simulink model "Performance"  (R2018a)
settings: Solver=ode113  StartTime=0.0  StopTime=20  FixedStep=0.0001  RelTol=1e-5  EnableMultiTasking=on
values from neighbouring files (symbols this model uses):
  d2r = pi/180    (= 0.0174532925199)    [init.m]
  Kr = Kq; Kr(3:4)=-Kq(3:4)    [init.m]
  r2d = 1/d2r    (= 57.2957795131)    [init.m]
  Wf = 20    [init.m]
undefined symbols (not defined in the file or in its folder): Aa, Av, Ba, Bv, Ca, Cv, Da, Dv, Kq, TVC

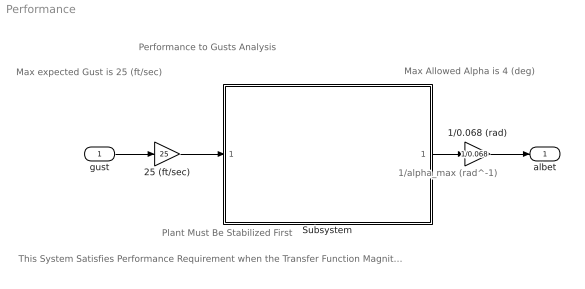
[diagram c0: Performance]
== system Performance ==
  note: Performance to Gusts Analysis
  note: Plant Must Be Stabilized First
  note: Max expected Gust is 25 (ft/sec)
  note: 1/alpha_max (rad^-1)
  note: This System Satisfies Performance Requirement when the Transfer Function Magnitude is Less than One at All Frequencies
  note: Max Allowed Alpha is 4 (deg)
  gust : Inport
  1/0.068 (rad) : Gain  Gain=1/0.068
  25 (ft/sec) : Gain  Gain=25
  Subsystem : Subsystem
  albet : Outport
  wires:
  gust/1 -> 25 (ft/sec)/1
  Subsystem/1(albet) -> 1/0.068 (rad)/1
  25 (ft/sec)/1 -> Subsystem/1(gust)
  1/0.068 (rad)/1 -> albet/1

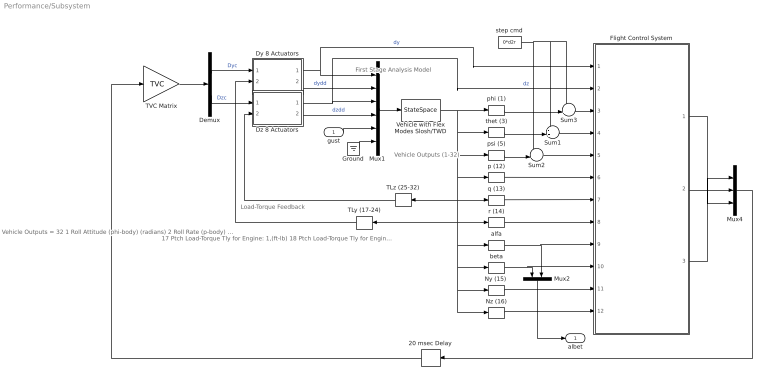
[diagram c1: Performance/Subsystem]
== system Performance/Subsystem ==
  note: First Stage Analysis Model
  note: Load-Torque Feedback
  note: 17 Ptch Load-Torque Tly for Engine: 1,(ft-lb) 18 Ptch Load-Torque Tly for Engine: 2,(ft-lb) 19 Ptch Load-Torque Tly for Engine: 3,(ft-lb) 20 Ptch Load-Torque Tly for Engine: 4,(ft-lb) 21 Ptch Load-Torque Tly for Engine: 5,(ft-lb) 22 Ptch Load-Torque Tly for Engine: 6,(ft-lb) 23 Ptch Load-Torque Tly for Engine: 7,(ft-lb) 24 Ptch Load-Torque Tly for Engine: 8,(ft-lb) 25 Yaw Load-Torque Tlz for Engine: 1,(ft-lb) 26 Yaw Load-Torque Tlz for Engine: 2,(ft-lb) 27 Yaw Load-Torque Tlz for Engine: 3,(ft-lb) 28 Yaw Load-Torque Tlz for Engine: 4,(ft-lb) 29 Yaw Load-Torque Tlz for Engine: 5,(ft-lb) 30 Yaw Load-Torque Tlz for Engine: 6,(ft-lb) 31 Yaw Load-Torque Tlz for Engine: 7,(ft-lb) 32 Yaw Load-Torque Tlz for Engine: 8,(ft-lb)
  note: Vehicle Outputs = 32 1 Roll Attitude (phi-body) (radians) 2 Roll Rate (p-body) (rad/sec) 3 Pitch Attitude (thet-bdy) (radians) 4 Pitch Rate (q-body) (rad/sec) 5 Yaw Attitude (psi-body) (radians) 6 Yaw Rate (r-body) (rad/sec) 7 Angle of attack, alfa, (radians) 8 Angle of sideslip, beta, (radian) 9 Change in Altitude, delta-h, (feet) 10 Forward Acceleration (V-dot) (ft/sec) 11 Cross Range Velocity (Vcr) (ft/sec) 12 Rate-Gyro # 1, Roll Rate (Body) (rad/sec) 13 Rate-Gyro # 2, Pitch Rate (Body) (rad/sec) 14 Rate-Gyro # 3, Yaw Rate (Body) (rad/sec) 15 Accelerom # 1, (along Y), (ft/sec^2) Translat. Accelerat. 16 Accelerom # 2, (along Z), (ft/sec^2) Translat. Accelerat.
  note: Vehicle Outputs (1-32)
  gust : Inport
  20 msec Delay : TransportDelay  DelayTime="[1  1  1]*0.02"  InitialOutput="[0  0  0]"  PadeOrder=2
  Demux : Demux  Outputs=[8, 8]
  Dy 8 Actuators : Subsystem
  Dz 8 Actuators : Subsystem
  Flight Control System : Subsystem
  Ground : Ground
  Mux1 : Mux  Inputs=[8, 8, 8, 8, 1, 38]
  Mux2 : Mux  Inputs=2
  Mux4 : Mux  Inputs=3
  "Ny (15) " : Selector  InputPortWidth=70  IndexOptions=Index vector (dialog)  Indices=[15]  OutputSizes=1
  Nz (16) : Selector  InputPortWidth=70  IndexOptions=Index vector (dialog)  Indices=[16]  OutputSizes=1
  Sum1 : Sum  Inputs=-+|
  Sum2 : Sum  Inputs=-+|
  Sum3 : Sum  Inputs=-+|
  TLy (17-24) : Selector  InputPortWidth=70  IndexOptions=Index vector (dialog)  Indices=[17:24]  OutputSizes=1
  TLz (25-32) : Selector  InputPortWidth=70  IndexOptions=Index vector (dialog)  Indices=[25:32]  OutputSizes=1
  TVC Matrix : Gain  Gain=TVC  Multiplication=Matrix(K*u)
  Vehicle with Flex Modes Slosh/TWD : StateSpace  A=Av  B=Bv  C=Cv  D=Dv  InitialCondition=0
  alfa : Selector  InputPortWidth=70  IndexOptions=Index vector (dialog)  Indices=[7]  OutputSizes=1
  beta : Selector  InputPortWidth=70  IndexOptions=Index vector (dialog)  Indices=[8]  OutputSizes=1
  p (12) : Selector  InputPortWidth=70  IndexOptions=Index vector (dialog)  Indices=[12]  OutputSizes=1
  phi (1) : Selector  InputPortWidth=70  IndexOptions=Index vector (dialog)  Indices=[1]  OutputSizes=1
  psi (5) : Selector  InputPortWidth=70  IndexOptions=Index vector (dialog)  Indices=[5]  OutputSizes=1
  q (13) : Selector  InputPortWidth=70  IndexOptions=Index vector (dialog)  Indices=[13]  OutputSizes=1
  r (14) : Selector  InputPortWidth=70  IndexOptions=Index vector (dialog)  Indices=[14]  OutputSizes=1
  step cmd : Constant  Value=0*d2r
  thet (3) : Selector  InputPortWidth=70  IndexOptions=Index vector (dialog)  Indices=[3]  OutputSizes=1
  albet : Outport
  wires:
  Mux1/1 -> Vehicle with Flex Modes Slosh/TWD/1
  Dz 8 Actuators/2(dzdd) -> Mux1/4  "dzdd"
  p (12)/1 -> Flight Control System/6(p)
  Vehicle with Flex Modes Slosh/TWD/1 -> TLz (25-32)/1, "Ny (15) "/1, Nz (16)/1, beta/1, alfa/1, TLy (17-24)/1, r (14)/1, q (13)/1, p (12)/1, psi (5)/1, thet (3)/1, phi (1)/1
  20 msec Delay/1 -> TVC Matrix/1
  TVC Matrix/1 -> Demux/1
  "Ny (15) "/1 -> Flight Control System/11(NY)
  Dz 8 Actuators/1(dz) -> Flight Control System/2(dz), Mux1/3  "dz"
  r (14)/1 -> Flight Control System/8(r)
  step cmd/1 -> Sum1/1, Sum3/1, Sum2/1
  TLy (17-24)/1 -> Dy 8 Actuators/2(TLy)
  TLz (25-32)/1 -> Dz 8 Actuators/2(TLz)
  alfa/1 -> Flight Control System/9(alfa), Mux2/2
  Flight Control System/2(DQ_tvc) -> Mux4/2
  Flight Control System/1(DP_tvc) -> Mux4/1
  Dy 8 Actuators/1(dy) -> Flight Control System/1(dy), Mux1/1  "dy"
  q (13)/1 -> Flight Control System/7(q)
  Dy 8 Actuators/2(dydd) -> Mux1/2  "dydd"
  beta/1 -> Flight Control System/10(beta), Mux2/1
  Flight Control System/3(DR_tvc) -> Mux4/3
  psi (5)/1 -> Sum2/2
  Demux/2 -> Dz 8 Actuators/1(dzc)  "Dzc"
  Sum2/1 -> Flight Control System/5(psi)
  Sum3/1 -> Flight Control System/3(phi)
  Sum1/1 -> Flight Control System/4(thet)
  Nz (16)/1 -> Flight Control System/12(NZ)
  thet (3)/1 -> Sum1/2
  Demux/1 -> Dy 8 Actuators/1(dyc)  "Dyc"
  phi (1)/1 -> Sum3/2
  Mux4/1 -> 20 msec Delay/1
  Ground/1 -> Mux1/6
  gust/1 -> Mux1/5
  Mux2/1 -> albet/1

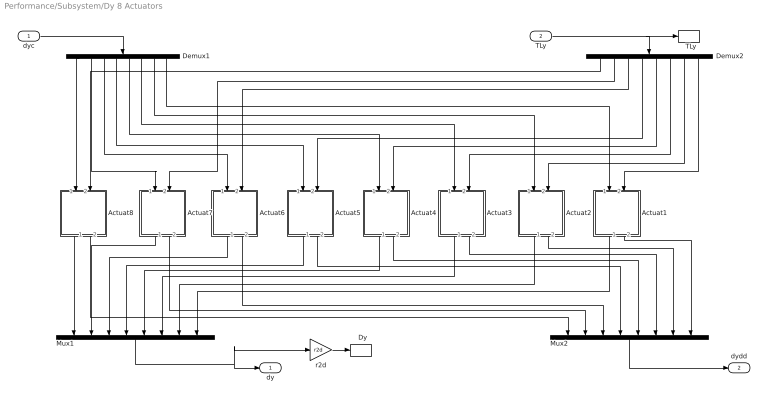
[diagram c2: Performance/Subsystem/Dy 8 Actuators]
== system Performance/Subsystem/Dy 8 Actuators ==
  dyc : Inport
  TLy : Inport  Port=2
  "  Dy" : ToWorkspace  VariableName=DY  SampleTime=-1
  "  TLy" : ToWorkspace  VariableName=TLy  SampleTime=-1
  Actuat1 : Subsystem
  Actuat2 : Subsystem
  Actuat3 : Subsystem
  Actuat4 : Subsystem
  Actuat5 : Subsystem
  Actuat6 : Subsystem
  Actuat7 : Subsystem
  Actuat8 : Subsystem
  Demux1 : Demux  Outputs=8
  Demux2 : Demux  Outputs=8
  Mux1 : Mux  Inputs=8
  Mux2 : Mux  Inputs=8
  r2d : Gain  Gain=r2d
  dy : Outport
  dydd : Outport  Port=2
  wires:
  TLy/1 -> "  TLy"/1, Demux2/1
  Mux2/1 -> dydd/1
  Actuat5/1(dout) -> Mux1/4
  Demux1/5 -> Actuat4/1(delin)
  Actuat3/2(ddot) -> Mux2/6
  Actuat8/1(dout) -> Mux1/1
  Demux1/4 -> Actuat5/1(delin)
  Actuat1/1(dout) -> Mux1/8
  Actuat4/2(ddot) -> Mux2/5
  Actuat4/1(dout) -> Mux1/5
  Demux2/4 -> Actuat5/2(TL)
  Demux2/6 -> Actuat3/2(TL)
  Demux2/7 -> Actuat2/2(TL)
  Actuat6/2(ddot) -> Mux2/3
  Demux2/2 -> Actuat7/2(TL)
  Actuat5/2(ddot) -> Mux2/4
  Demux1/3 -> Actuat6/1(delin)
  Actuat2/2(ddot) -> Mux2/7
  Actuat8/2(ddot) -> Mux2/1
  dyc/1 -> Demux1/1
  Mux1/1 -> r2d/1, dy/1
  Actuat1/2(ddot) -> Mux2/8
  Actuat7/2(ddot) -> Mux2/2
  Demux1/2 -> Actuat7/1(delin)
  Demux1/7 -> Actuat2/1(delin)
  Demux1/8 -> Actuat1/1(delin)
  Actuat7/1(dout) -> Mux1/2
  Demux2/5 -> Actuat4/2(TL)
  Demux1/1 -> Actuat8/1(delin)
  Demux2/1 -> Actuat8/2(TL)
  Actuat2/1(dout) -> Mux1/7
  Demux2/8 -> Actuat1/2(TL)
  Demux2/3 -> Actuat6/2(TL)
  Actuat3/1(dout) -> Mux1/6
  Actuat6/1(dout) -> Mux1/3
  Demux1/6 -> Actuat3/1(delin)
  r2d/1 -> "  Dy"/1

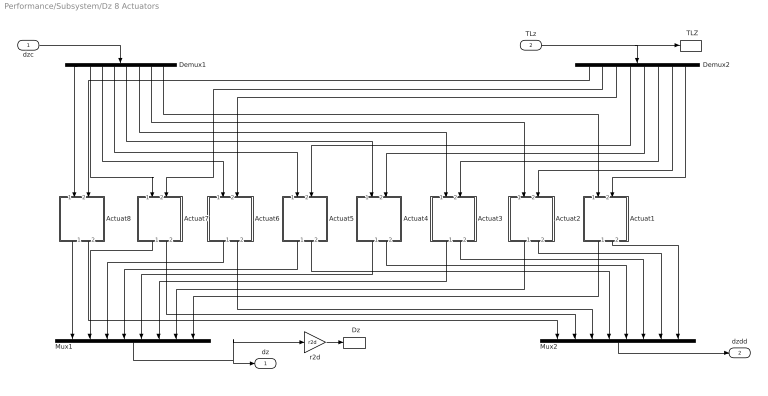
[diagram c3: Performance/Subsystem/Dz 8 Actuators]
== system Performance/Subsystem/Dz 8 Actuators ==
  dzc : Inport
  TLz : Inport  Port=2
  "  Dz" : ToWorkspace  VariableName=DZ  SampleTime=-1
  "  TLZ" : ToWorkspace  VariableName=TLz  SampleTime=-1
  Actuat1 : Subsystem
  Actuat2 : Subsystem
  Actuat3 : Subsystem
  Actuat4 : Subsystem
  Actuat5 : Subsystem
  Actuat6 : Subsystem
  Actuat7 : Subsystem
  Actuat8 : Subsystem
  Demux1 : Demux  Outputs=8
  Demux2 : Demux  Outputs=8
  Mux1 : Mux  Inputs=8
  Mux2 : Mux  Inputs=8
  r2d : Gain  Gain=r2d
  dz : Outport
  dzdd : Outport  Port=2
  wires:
  TLz/1 -> "  TLZ"/1, Demux2/1
  Mux2/1 -> dzdd/1
  Actuat5/1(dout) -> Mux1/4
  Demux1/5 -> Actuat4/1(delin)
  Actuat3/2(ddot) -> Mux2/6
  Actuat8/1(dout) -> Mux1/1
  Demux1/4 -> Actuat5/1(delin)
  Actuat1/1(dout) -> Mux1/8
  Actuat4/2(ddot) -> Mux2/5
  Actuat4/1(dout) -> Mux1/5
  Demux2/4 -> Actuat5/2(TL)
  Demux2/6 -> Actuat3/2(TL)
  Demux2/7 -> Actuat2/2(TL)
  Actuat6/2(ddot) -> Mux2/3
  Demux2/2 -> Actuat7/2(TL)
  Actuat5/2(ddot) -> Mux2/4
  Demux1/3 -> Actuat6/1(delin)
  Actuat2/2(ddot) -> Mux2/7
  Actuat8/2(ddot) -> Mux2/1
  dzc/1 -> Demux1/1
  Mux1/1 -> r2d/1, dz/1
  Actuat1/2(ddot) -> Mux2/8
  Actuat7/2(ddot) -> Mux2/2
  Demux1/2 -> Actuat7/1(delin)
  Demux1/7 -> Actuat2/1(delin)
  Demux1/8 -> Actuat1/1(delin)
  Actuat7/1(dout) -> Mux1/2
  Demux2/5 -> Actuat4/2(TL)
  Demux1/1 -> Actuat8/1(delin)
  Demux2/1 -> Actuat8/2(TL)
  Actuat2/1(dout) -> Mux1/7
  Demux2/8 -> Actuat1/2(TL)
  Demux2/3 -> Actuat6/2(TL)
  Actuat3/1(dout) -> Mux1/6
  Actuat6/1(dout) -> Mux1/3
  Demux1/6 -> Actuat3/1(delin)
  r2d/1 -> "  Dz"/1

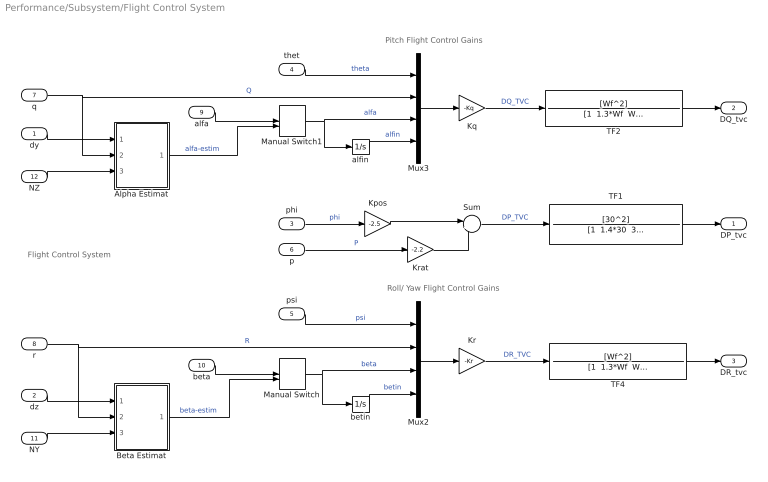
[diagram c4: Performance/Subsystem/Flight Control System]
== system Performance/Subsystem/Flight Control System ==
  note: Flight Control System
  note: Roll/ Yaw Flight Control Gains
  note: Pitch Flight Control Gains
  dy : Inport
  dz : Inport  Port=2
  phi : Inport  Port=3
  thet : Inport  Port=4
  psi : Inport  Port=5
  p : Inport  Port=6
  q : Inport  Port=7
  r : Inport  Port=8
  alfa : Inport  Port=9
  beta : Inport  Port=10
  NY : Inport  Port=11
  NZ : Inport  Port=12
  Alpha Estimat : Subsystem
  Beta Estimat : Subsystem
  Kpos : Gain  Gain=-2.5  Multiplication=Matrix(K*u)
  Kq : Gain  Gain=-Kq  Multiplication=Matrix(K*u)
  Kr : Gain  Gain=-Kr  Multiplication=Matrix(K*u)
  Krat : Gain  Gain=-2.2  Multiplication=Matrix(K*u)
  Manual Switch : ManualSwitch  CurrentSetting=0
  Manual Switch1 : ManualSwitch  CurrentSetting=0
  Mux2 : Mux
  Mux3 : Mux
  Sum : Sum  Inputs=|++
  TF1 : TransferFcn  Numerator=[30^2]  Denominator="[1  1.4*30  30^2]"
  TF2 : TransferFcn  Numerator=[Wf^2]  Denominator="[1  1.3*Wf  Wf^2]"
  TF4 : TransferFcn  Numerator=[Wf^2]  Denominator="[1  1.3*Wf  Wf^2]"
  alfin : Integrator
  betin : Integrator
  DP_tvc : Outport
  DQ_tvc : Outport  Port=2
  DR_tvc : Outport  Port=3
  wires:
  TF4/1 -> DR_tvc/1
  Kr/1 -> TF4/1  "DR_TVC"
  TF2/1 -> DQ_tvc/1
  TF1/1 -> DP_tvc/1
  Mux2/1 -> Kr/1
  phi/1 -> Kpos/1  "phi"
  p/1 -> Krat/1  "P"
  Krat/1 -> Sum/2
  Sum/1 -> TF1/1  "DP_TVC"
  Kpos/1 -> Sum/1
  Mux3/1 -> Kq/1
  dz/1 -> Beta Estimat/1(dz)
  dy/1 -> Alpha Estimat/1(dy)
  Beta Estimat/1(betest) -> Manual Switch/2  "beta-estim"
  NY/1 -> Beta Estimat/3(Ydd)
  NZ/1 -> Alpha Estimat/3(Zdd)
  Kq/1 -> TF2/1  "DQ_TVC"
  thet/1 -> Mux3/1  "theta"
  alfin/1 -> Mux3/4  "alfin"
  r/1 -> Beta Estimat/2(r), Mux2/2  "R"
  q/1 -> Mux3/2, Alpha Estimat/2(q)  "Q"
  betin/1 -> Mux2/4  "betin"
  psi/1 -> Mux2/1  "psi"
  Manual Switch/1 -> Mux2/3, betin/1  "beta"
  beta/1 -> Manual Switch/1
  Manual Switch1/1 -> alfin/1, Mux3/3  "alfa"
  alfa/1 -> Manual Switch1/1
  Alpha Estimat/1(alfest) -> Manual Switch1/2  "alfa-estim"

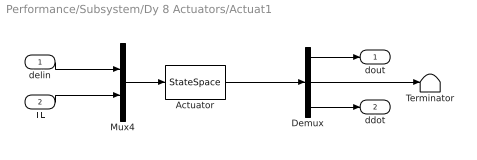
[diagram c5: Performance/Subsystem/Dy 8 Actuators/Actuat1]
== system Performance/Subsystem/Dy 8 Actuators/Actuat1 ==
  delin : Inport
  TL : Inport  Port=2
  Actuator : StateSpace  A=Aa  B=Ba  C=Ca  D=Da  InitialCondition=0
  Demux : Demux  Outputs=3
  Mux4 : Mux  Inputs=2
  Terminator : Terminator
  dout : Outport
  ddot : Outport  Port=2
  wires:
  Demux/3 -> ddot/1
  TL/1 -> Mux4/2
  Mux4/1 -> Actuator/1
  Actuator/1 -> Demux/1
  delin/1 -> Mux4/1
  Demux/1 -> dout/1
  Demux/2 -> Terminator/1

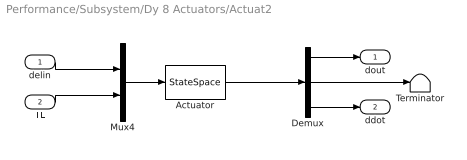
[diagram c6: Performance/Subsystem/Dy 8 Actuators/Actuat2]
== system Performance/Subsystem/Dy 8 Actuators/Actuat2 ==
  delin : Inport
  TL : Inport  Port=2
  Actuator : StateSpace  A=Aa  B=Ba  C=Ca  D=Da  InitialCondition=0
  Demux : Demux  Outputs=3
  Mux4 : Mux  Inputs=2
  Terminator : Terminator
  dout : Outport
  ddot : Outport  Port=2
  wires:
  Demux/3 -> ddot/1
  TL/1 -> Mux4/2
  Mux4/1 -> Actuator/1
  Actuator/1 -> Demux/1
  delin/1 -> Mux4/1
  Demux/1 -> dout/1
  Demux/2 -> Terminator/1

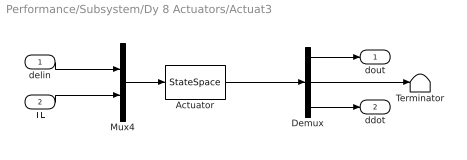
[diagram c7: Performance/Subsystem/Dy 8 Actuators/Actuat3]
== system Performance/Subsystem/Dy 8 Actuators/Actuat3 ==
  delin : Inport
  TL : Inport  Port=2
  Actuator : StateSpace  A=Aa  B=Ba  C=Ca  D=Da  InitialCondition=0
  Demux : Demux  Outputs=3
  Mux4 : Mux  Inputs=2
  Terminator : Terminator
  dout : Outport
  ddot : Outport  Port=2
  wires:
  Demux/3 -> ddot/1
  TL/1 -> Mux4/2
  Mux4/1 -> Actuator/1
  Actuator/1 -> Demux/1
  delin/1 -> Mux4/1
  Demux/1 -> dout/1
  Demux/2 -> Terminator/1

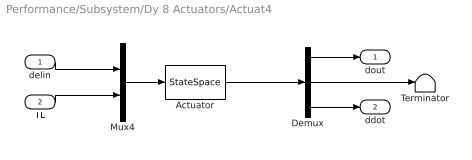
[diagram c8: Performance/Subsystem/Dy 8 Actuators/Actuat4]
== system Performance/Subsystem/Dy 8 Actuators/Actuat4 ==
  delin : Inport
  TL : Inport  Port=2
  Actuator : StateSpace  A=Aa  B=Ba  C=Ca  D=Da  InitialCondition=0
  Demux : Demux  Outputs=3
  Mux4 : Mux  Inputs=2
  Terminator : Terminator
  dout : Outport
  ddot : Outport  Port=2
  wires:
  Demux/3 -> ddot/1
  TL/1 -> Mux4/2
  Mux4/1 -> Actuator/1
  Actuator/1 -> Demux/1
  delin/1 -> Mux4/1
  Demux/1 -> dout/1
  Demux/2 -> Terminator/1

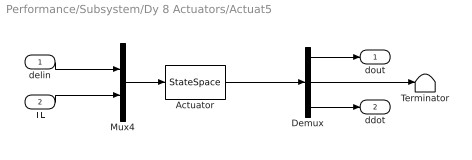
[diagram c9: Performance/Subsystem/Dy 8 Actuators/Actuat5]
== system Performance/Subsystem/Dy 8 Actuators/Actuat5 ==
  delin : Inport
  TL : Inport  Port=2
  Actuator : StateSpace  A=Aa  B=Ba  C=Ca  D=Da  InitialCondition=0
  Demux : Demux  Outputs=3
  Mux4 : Mux  Inputs=2
  Terminator : Terminator
  dout : Outport
  ddot : Outport  Port=2
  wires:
  Demux/3 -> ddot/1
  TL/1 -> Mux4/2
  Mux4/1 -> Actuator/1
  Actuator/1 -> Demux/1
  delin/1 -> Mux4/1
  Demux/1 -> dout/1
  Demux/2 -> Terminator/1

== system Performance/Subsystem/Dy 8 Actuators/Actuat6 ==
  delin : Inport
  TL : Inport  Port=2
  Actuator : StateSpace  A=Aa  B=Ba  C=Ca  D=Da  InitialCondition=0
  Demux : Demux  Outputs=3
  Mux4 : Mux  Inputs=2
  Terminator : Terminator
  dout : Outport
  ddot : Outport  Port=2
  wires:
  Demux/3 -> ddot/1
  TL/1 -> Mux4/2
  Mux4/1 -> Actuator/1
  Actuator/1 -> Demux/1
  delin/1 -> Mux4/1
  Demux/1 -> dout/1
  Demux/2 -> Terminator/1

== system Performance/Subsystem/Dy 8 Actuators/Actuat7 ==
  delin : Inport
  TL : Inport  Port=2
  Actuator : StateSpace  A=Aa  B=Ba  C=Ca  D=Da  InitialCondition=0
  Demux : Demux  Outputs=3
  Mux4 : Mux  Inputs=2
  Terminator : Terminator
  dout : Outport
  ddot : Outport  Port=2
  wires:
  Demux/3 -> ddot/1
  TL/1 -> Mux4/2
  Mux4/1 -> Actuator/1
  Actuator/1 -> Demux/1
  delin/1 -> Mux4/1
  Demux/1 -> dout/1
  Demux/2 -> Terminator/1

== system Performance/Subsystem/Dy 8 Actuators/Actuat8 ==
  delin : Inport
  TL : Inport  Port=2
  Actuator : StateSpace  A=Aa  B=Ba  C=Ca  D=Da  InitialCondition=0
  Demux : Demux  Outputs=3
  Mux4 : Mux  Inputs=2
  Terminator : Terminator
  dout : Outport
  ddot : Outport  Port=2
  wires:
  Demux/3 -> ddot/1
  TL/1 -> Mux4/2
  Mux4/1 -> Actuator/1
  Actuator/1 -> Demux/1
  delin/1 -> Mux4/1
  Demux/1 -> dout/1
  Demux/2 -> Terminator/1

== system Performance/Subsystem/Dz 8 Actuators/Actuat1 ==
  delin : Inport
  TL : Inport  Port=2
  Actuator : StateSpace  A=Aa  B=Ba  C=Ca  D=Da  InitialCondition=0
  Demux : Demux  Outputs=3
  Mux4 : Mux  Inputs=2
  Terminator : Terminator
  dout : Outport
  ddot : Outport  Port=2
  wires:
  Demux/3 -> ddot/1
  TL/1 -> Mux4/2
  Mux4/1 -> Actuator/1
  Actuator/1 -> Demux/1
  delin/1 -> Mux4/1
  Demux/1 -> dout/1
  Demux/2 -> Terminator/1

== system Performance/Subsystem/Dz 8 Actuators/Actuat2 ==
  delin : Inport
  TL : Inport  Port=2
  Actuator : StateSpace  A=Aa  B=Ba  C=Ca  D=Da  InitialCondition=0
  Demux : Demux  Outputs=3
  Mux4 : Mux  Inputs=2
  Terminator : Terminator
  dout : Outport
  ddot : Outport  Port=2
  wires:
  Demux/3 -> ddot/1
  TL/1 -> Mux4/2
  Mux4/1 -> Actuator/1
  Actuator/1 -> Demux/1
  delin/1 -> Mux4/1
  Demux/1 -> dout/1
  Demux/2 -> Terminator/1

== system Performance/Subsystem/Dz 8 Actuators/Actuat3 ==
  delin : Inport
  TL : Inport  Port=2
  Actuator : StateSpace  A=Aa  B=Ba  C=Ca  D=Da  InitialCondition=0
  Demux : Demux  Outputs=3
  Mux4 : Mux  Inputs=2
  Terminator : Terminator
  dout : Outport
  ddot : Outport  Port=2
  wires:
  Demux/3 -> ddot/1
  TL/1 -> Mux4/2
  Mux4/1 -> Actuator/1
  Actuator/1 -> Demux/1
  delin/1 -> Mux4/1
  Demux/1 -> dout/1
  Demux/2 -> Terminator/1

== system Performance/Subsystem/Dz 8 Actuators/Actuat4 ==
  delin : Inport
  TL : Inport  Port=2
  Actuator : StateSpace  A=Aa  B=Ba  C=Ca  D=Da  InitialCondition=0
  Demux : Demux  Outputs=3
  Mux4 : Mux  Inputs=2
  Terminator : Terminator
  dout : Outport
  ddot : Outport  Port=2
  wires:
  Demux/3 -> ddot/1
  TL/1 -> Mux4/2
  Mux4/1 -> Actuator/1
  Actuator/1 -> Demux/1
  delin/1 -> Mux4/1
  Demux/1 -> dout/1
  Demux/2 -> Terminator/1

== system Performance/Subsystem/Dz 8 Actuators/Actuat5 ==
  delin : Inport
  TL : Inport  Port=2
  Actuator : StateSpace  A=Aa  B=Ba  C=Ca  D=Da  InitialCondition=0
  Demux : Demux  Outputs=3
  Mux4 : Mux  Inputs=2
  Terminator : Terminator
  dout : Outport
  ddot : Outport  Port=2
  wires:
  Demux/3 -> ddot/1
  TL/1 -> Mux4/2
  Mux4/1 -> Actuator/1
  Actuator/1 -> Demux/1
  delin/1 -> Mux4/1
  Demux/1 -> dout/1
  Demux/2 -> Terminator/1

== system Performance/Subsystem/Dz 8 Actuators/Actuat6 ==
  delin : Inport
  TL : Inport  Port=2
  Actuator : StateSpace  A=Aa  B=Ba  C=Ca  D=Da  InitialCondition=0
  Demux : Demux  Outputs=3
  Mux4 : Mux  Inputs=2
  Terminator : Terminator
  dout : Outport
  ddot : Outport  Port=2
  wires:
  Demux/3 -> ddot/1
  TL/1 -> Mux4/2
  Mux4/1 -> Actuator/1
  Actuator/1 -> Demux/1
  delin/1 -> Mux4/1
  Demux/1 -> dout/1
  Demux/2 -> Terminator/1

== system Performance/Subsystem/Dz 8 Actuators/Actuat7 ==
  delin : Inport
  TL : Inport  Port=2
  Actuator : StateSpace  A=Aa  B=Ba  C=Ca  D=Da  InitialCondition=0
  Demux : Demux  Outputs=3
  Mux4 : Mux  Inputs=2
  Terminator : Terminator
  dout : Outport
  ddot : Outport  Port=2
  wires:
  Demux/3 -> ddot/1
  TL/1 -> Mux4/2
  Mux4/1 -> Actuator/1
  Actuator/1 -> Demux/1
  delin/1 -> Mux4/1
  Demux/1 -> dout/1
  Demux/2 -> Terminator/1

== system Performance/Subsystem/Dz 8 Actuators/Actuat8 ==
  delin : Inport
  TL : Inport  Port=2
  Actuator : StateSpace  A=Aa  B=Ba  C=Ca  D=Da  InitialCondition=0
  Demux : Demux  Outputs=3
  Mux4 : Mux  Inputs=2
  Terminator : Terminator
  dout : Outport
  ddot : Outport  Port=2
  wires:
  Demux/3 -> ddot/1
  TL/1 -> Mux4/2
  Mux4/1 -> Actuator/1
  Actuator/1 -> Demux/1
  delin/1 -> Mux4/1
  Demux/1 -> dout/1
  Demux/2 -> Terminator/1

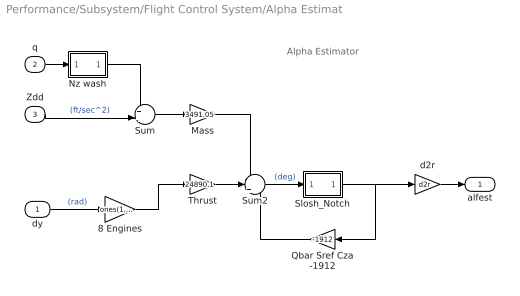
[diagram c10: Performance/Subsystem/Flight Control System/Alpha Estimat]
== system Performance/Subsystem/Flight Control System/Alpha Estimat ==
  note: Alpha Estimator
  dy : Inport
  q : Inport  Port=2
  Zdd : Inport  Port=3
  8 Engines : Gain  Gain=ones(1,8)  Multiplication=Matrix(K*u) (u vector)
  Mass : Gain  Gain=3491.05
  Nz wash : Subsystem
  Qbar Sref Cza -1912 : Gain  Gain=-1912
  Slosh_Notch : Subsystem
  Sum : Sum  Inputs=++|
  Sum2 : Sum  Inputs=--+
  Thrust : Gain  Gain=24890.1
  d2r : Gain  Gain=d2r
  alfest : Outport
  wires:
  8 Engines/1 -> Thrust/1
  Thrust/1 -> Sum2/2
  Mass/1 -> Sum2/1
  Slosh_Notch/1(ou) -> Qbar Sref Cza -1912/1, d2r/1
  Nz wash/1(ou) -> Sum/1
  Sum2/1 -> Slosh_Notch/1(in)  "(deg)"
  Qbar Sref Cza -1912/1 -> Sum2/3
  Zdd/1 -> Sum/2  "(ft/sec^2)"
  d2r/1 -> alfest/1
  q/1 -> Nz wash/1(in)
  Sum/1 -> Mass/1
  dy/1 -> 8 Engines/1  "(rad)"

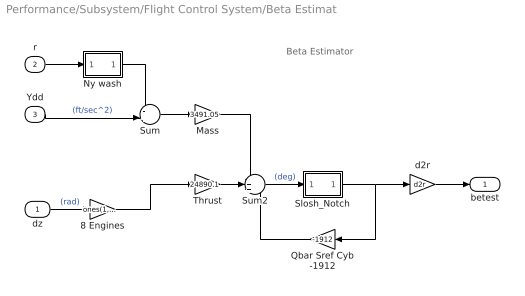
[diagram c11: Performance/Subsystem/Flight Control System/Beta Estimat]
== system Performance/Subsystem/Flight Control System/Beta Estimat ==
  note: Beta Estimator
  dz : Inport
  r : Inport  Port=2
  Ydd : Inport  Port=3
  8 Engines : Gain  Gain=ones(1,8)  Multiplication=Matrix(K*u) (u vector)
  Mass : Gain  Gain=3491.05
  Ny wash : Subsystem
  Qbar Sref Cyb -1912 : Gain  Gain=-1912
  Slosh_Notch : Subsystem
  Sum : Sum  Inputs=-+|
  Sum2 : Sum  Inputs=-++
  Thrust : Gain  Gain=24890.1
  d2r : Gain  Gain=d2r
  betest : Outport
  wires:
  8 Engines/1 -> Thrust/1
  dz/1 -> 8 Engines/1  "(rad)"
  Slosh_Notch/1(ou) -> d2r/1, Qbar Sref Cyb -1912/1
  Ny wash/1(ou) -> Sum/1
  Sum2/1 -> Slosh_Notch/1(in)  "(deg)"
  Qbar Sref Cyb -1912/1 -> Sum2/3
  Ydd/1 -> Sum/2  "(ft/sec^2)"
  Mass/1 -> Sum2/1
  d2r/1 -> betest/1
  Thrust/1 -> Sum2/2
  r/1 -> Ny wash/1(in)
  Sum/1 -> Mass/1

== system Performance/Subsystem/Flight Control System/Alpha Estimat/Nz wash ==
  in : Inport
  3 : Gain  Gain=19
  Transfer Fcn : TransferFcn  Numerator="[1  0]"  Denominator="[0.015  1]"
  ou : Outport
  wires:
  3/1 -> ou/1
  Transfer Fcn/1 -> 3/1
  in/1 -> Transfer Fcn/1

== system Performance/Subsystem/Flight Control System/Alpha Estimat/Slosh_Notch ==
  in : Inport
  0.1 : Gain  Gain=0.00035
  Int1 : Integrator
  Transfer Fcn2 : TransferFcn  Numerator="[1 0.016*4.4  4.38^2]"  Denominator="[1  0.32*4.4  4.38^2]"
  ou : Outport
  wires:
  Int1/1 -> ou/1
  0.1/1 -> Transfer Fcn2/1
  Transfer Fcn2/1 -> Int1/1
  in/1 -> 0.1/1

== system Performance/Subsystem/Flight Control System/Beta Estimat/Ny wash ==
  in : Inport
  3 : Gain  Gain=19
  Transfer Fcn1 : TransferFcn  Numerator="[1  0]"  Denominator="[0.015  1]"
  ou : Outport
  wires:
  3/1 -> ou/1
  Transfer Fcn1/1 -> 3/1
  in/1 -> Transfer Fcn1/1

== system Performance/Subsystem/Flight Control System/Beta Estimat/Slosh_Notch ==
  in : Inport
  0.1 : Gain  Gain=0.00035
  Int1 : Integrator
  Transfer Fcn2 : TransferFcn  Numerator="[1 0.016*4.4  4.38^2]"  Denominator="[1  0.32*4.4  4.38^2]"
  ou : Outport
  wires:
  Transfer Fcn2/1 -> Int1/1
  0.1/1 -> Transfer Fcn2/1
  Int1/1 -> ou/1
  in/1 -> 0.1/1
